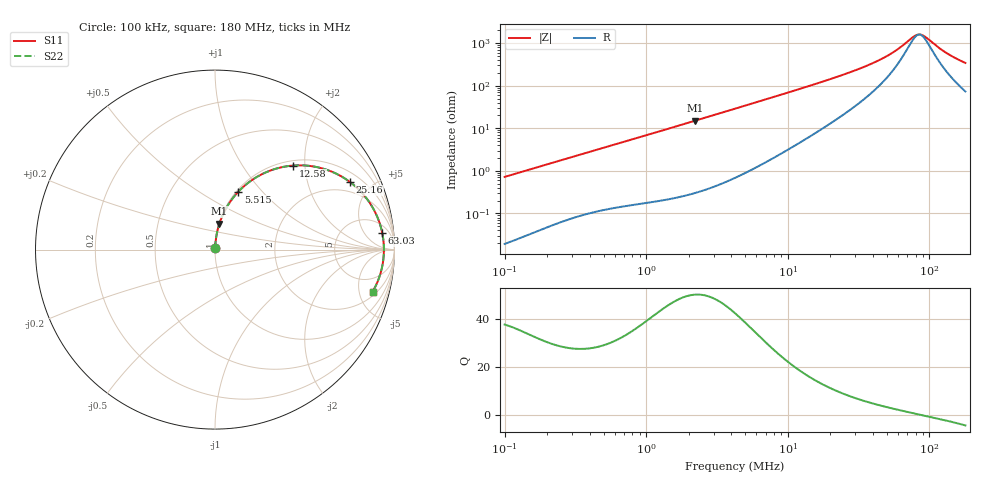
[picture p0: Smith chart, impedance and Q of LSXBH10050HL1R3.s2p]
! LSXBH10050HL1R3  S-PARAMETER MODEL  ( General Type )
! Model Generated by TAIYO YUDEN Corporation (http://www.ty-top.com)
! Version 3.0
! TAIYO YUDEN Control No. 180118NI43SB-FBB
! Copyright(c) 2007 TAIYO YUDEN CO.,LTD. All Rights Reserved.
! Product Description (link to TY-COMPAS)
! https://ds.yuden.co.jp/TYCOMPAS/or/detail?pn=LSXBH10050HL1R3N&u=M
! Products Name : Inductors
! Characteristics :
!  Inductance : 1.3 uH , SRF(min) : 53 MHz , DC Resistance(max) : 0.00884 Ohm
!  Rated Current : Saturation :11000 mA , Temp Rise : 9000 mA (40 degC)
!  Case Size : 10.0 x 9.8 / 0.394 x 0.386 [mm/inch] , Thickness : 5 / 0.197 [mm/inch]
!  (Conditions: Temperature = 25 degC , DC Bias Current/Voltage = 0A / 0V)
! External Node Assignments :
!  1  o---GGG---o  2
! GND o---------o GND
! Frequency Range : 0.1MHz  -  180.004543MHz  [ 402 STEP ]
# MHz S RI R 50
! Freq[MHz].  S11 Real  S11 Imag  S21 Real  S21 Imag  S12 Real  S12 Imag  S22 Real  S22 Imag
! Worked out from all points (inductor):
!   401 points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, 100 kHz to 180 MHz, reference 50 ohm
!   read as one part in series: L = 1.14 uH near 103.8 kHz
!   highest Q = 50 at 2.202 MHz (marker M1), where L = 1.08 uH
!   self-resonance near 85.02 MHz
!   S11 on the Smith chart (normalised r, x): 100 kHz: 1.00, +0.01; 5.515 MHz: 1.02, +0.75; 12.58 MHz: 1.10, +1.74; 25.16 MHz: 1.43, +3.69; 63.03 MHz: 9, +14; 180 MHz: 2.46, -6.68
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0.1  0.000243 0.00719  0.9998 -0.00719  0.9998 -0.00719  0.000243 0.00719
0.350962  0.0015 0.0245  0.9985 -0.0245  0.9985 -0.0245  0.0015 0.0245
1.231743  0.00889 0.0829  0.9911 -0.0829  0.9911 -0.0829  0.00889 0.0829
2.201935  0.0246 0.1453  0.9754 -0.1453  0.9754 -0.1453  0.0246 0.1453
4.322947  0.0848 0.2668  0.9152 -0.2668  0.9152 -0.2668  0.0848 0.2668
5.515395  0.1301 0.3228  0.8699 -0.3228  0.8699 -0.3228  0.1301 0.3228
8.174836  0.246 0.4122  0.754 -0.4122  0.754 -0.4122  0.246 0.4122
12.57934  0.4344 0.4683  0.5656 -0.4683  0.5656 -0.4683  0.4344 0.4683
14.89024  0.5176 0.4674  0.4824 -0.4674  0.4824 -0.4674  0.5176 0.4674
18.99759  0.6345 0.4405  0.3655 -0.4405  0.3655 -0.4405  0.6345 0.4405
25.16353  0.7504 0.3778  0.2496 -0.3778  0.2496 -0.3778  0.7504 0.3778
38.0025  0.8668 0.2535  0.1332 -0.2535  0.1332 -0.2535  0.8668 0.2535
52.25907  0.916 0.1515  0.084 -0.1515  0.084 -0.1515  0.916 0.1515
63.02949  0.9319 0.0925  0.0681 -0.0925  0.0681 -0.0925  0.9319 0.0925
77.45761  0.9402 0.0287  0.0598 -0.0287  0.0598 -0.0287  0.9402 0.0287
81.93674  0.941 0.0114  0.059 -0.0114  0.059 -0.0114  0.941 0.0114
86.6749  0.9411 -0.00591  0.0589 0.00591  0.0589 0.00591  0.9411 -0.00591
93.42136  0.9402 -0.029  0.0598 0.029  0.0598 0.029  0.9402 -0.029
114.8065  0.9319 -0.0928  0.0681 0.0928  0.0681 0.0928  0.9319 -0.0928
133.3743  0.9198 -0.14  0.0802 0.14  0.0802 0.14  0.9198 -0.14
157.876  0.8994 -0.1937  0.1006 0.1937  0.1006 0.1937  0.8994 -0.1937
180.0045  0.8777 -0.2359  0.1223 0.2359  0.1223 0.2359  0.8777 -0.2359
